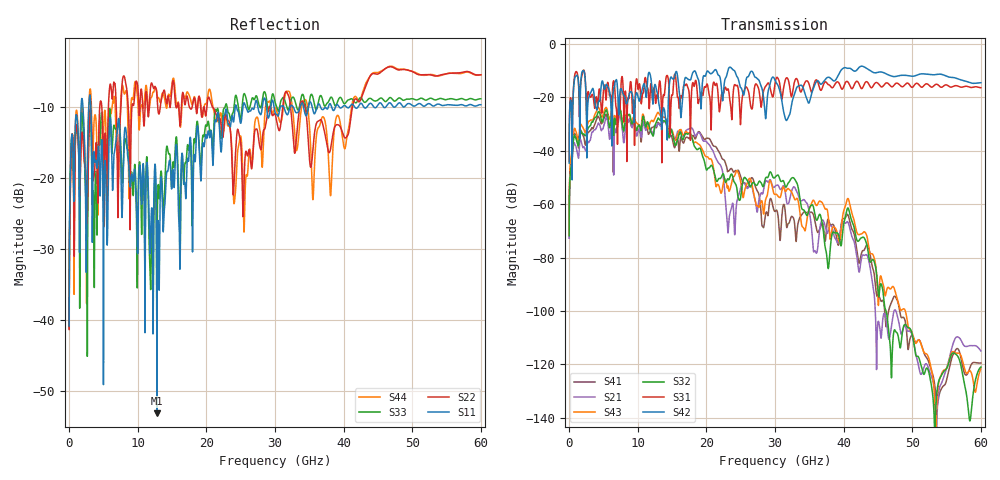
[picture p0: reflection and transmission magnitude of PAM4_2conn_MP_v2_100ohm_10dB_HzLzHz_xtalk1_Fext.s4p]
! Info: Touchstone file created by Circ.  Input file=FAB50GbE_2conn_Midplane_Examax_Topo2_v2_100ohm_10dB_HzLzHz.circ
# Hz S RI R 50
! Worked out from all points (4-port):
!   6000 points, 10 MHz to 60 GHz, reference 50 ohm
!   strongest paths, dB at 10 MHz, 15.01 GHz, 30.01 GHz, 45.01 GHz, 60 GHz:
!     S42: -44.6, -12.9, -13.6, -10.6, -14.5
!     S31: -43.9, -19.0, -14.7, -14.8, -16.4
!     S32: -71.9, -33.1, -50.0, -92.3, -121.0
!     S43: -71.5, -32.7, -56.4, -95.9, -121.5
!     S21: -72.7, -32.4, -53.4, -104.2, -115.0
!     S41: -67.7, -35.2, -62.7, -94.4, -119.5
!   lowest |S11| = -53.1 dB at 12.82 GHz (marker M1), VSWR 1.00, Z = 49.9 + j0.207 ohm
!   |S11| at or under -10 dB: start of sweep to 1.754 GHz; 3.171 GHz to 24.2 GHz (21.03 GHz wide, 154 % of centre); 25.77 GHz to 27.01 GHz (1.238 GHz wide, 4.69 % of centre)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
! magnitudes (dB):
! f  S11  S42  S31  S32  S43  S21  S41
! 10 MHz  -40.8  -44.6  -43.9  -71.9  -71.5  -72.7  -67.7
! 860 MHz  -14.0  -12.6  -11.3  -34.6  -31.7  -37.7  -33.6
! 12.82 GHz  -53.1  -17.9  -19.1  -28.7  -26.1  -30.6  -30.6
! 20.34 GHz  -13.5  -10.4  -18.1  -46.5  -42.8  -37.5  -35.4
! 23.19 GHz  -12.4  -9.5  -16.9  -50.7  -53.9  -70.0  -47.6
! 37.72 GHz  -10.2  -12.5  -15.2  -83.7  -63.5  -70.4  -65.7
! 60 GHz  -9.7  -14.5  -16.4  -121.0  -121.5  -115.0  -119.5
